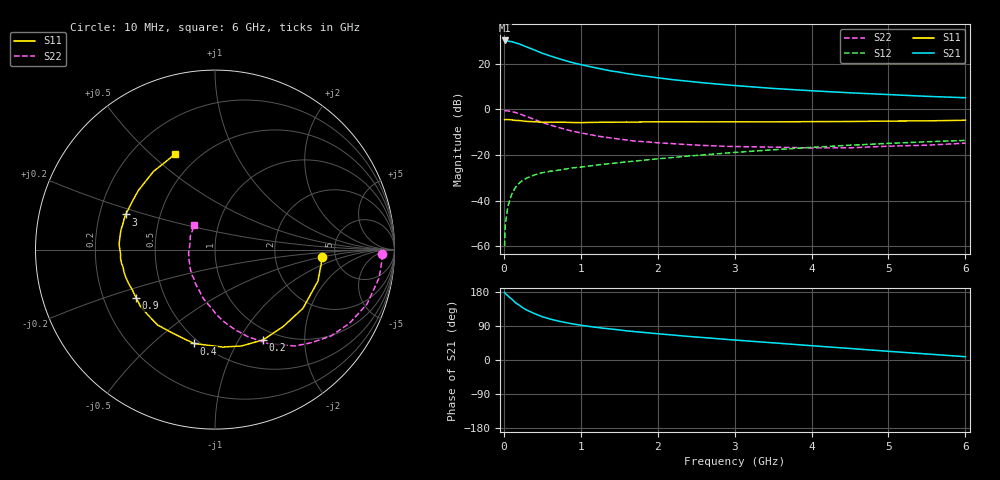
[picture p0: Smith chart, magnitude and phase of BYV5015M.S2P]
! SIEMENS Small Signal Semiconductors
! BFY420
! Si NPN RF SIEGET Grounded Emitter Transistor in MICRO-X
! VCE = 0.5 V  IC = 15 mA
! Common Emitter S-Parameters:  October  1996
# GHz  S  MA  R  50
!  f  S11  S21  S12  S22
! GHz  MAG  ANG  MAG  ANG  MAG  ANG  MAG  ANG
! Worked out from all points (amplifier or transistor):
!   36 points, 10 MHz to 6 GHz, reference 50 ohm
!   highest |S21| = 30.2 dB at 10 MHz (marker M1)
!   |S21| within 3 dB of that: start of sweep to 308.1 MHz
!   unconditionally stable (mu >= 1): start of sweep to 11.19 MHz; 1.834 GHz to end of sweep
!   at 250 MHz: K = 0.27, MSG = 29.5 dB, |S12| = -31.0 dB
!   at 1.4 GHz: K = 0.91, MSG = 20.3 dB, |S12| = -23.7 dB
!   at 6 GHz: K = 1.12, MAG = 7.2 dB, |S12| = -13.6 dB
!   S11 on the Smith chart (normalised r, x): 10 MHz: 3.90, -0.51; 200 MHz: 0.85, -1.27; 400 MHz: 0.47, -0.69; 900 MHz: 0.34, -0.25; 3 GHz: 0.31, +0.17; 6 GHz: 0.37, +0.60
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0.01  0.5979 -4.0  32.53 178.8  0.001 94.5  0.9324 -1.6
0.02  0.5971 -7.4  32.47 175.5  0.003 89.2  0.9322 -3.6
0.05  0.5998 -17.0  31.54 169.8  0.0072 84.0  0.9281 -9.7
0.1  0.5893 -33.8  30.66 161.1  0.0135 76.4  0.8996 -19.7
0.15  0.5727 -48.4  28.92 151.6  0.0194 68.9  0.8545 -28.7
0.2  0.5701 -62.0  27.28 144.6  0.0242 65.1  0.8059 -36.7
0.25  0.5568 -74.7  25.23 137.3  0.0281 59.8  0.7458 -44.1
0.3  0.5448 -85.5  23.31 131.5  0.0314 56.9  0.6972 -50.4
0.4  0.5362 -102.7  20 122.3  0.0367 51.9  0.5977 -60.9
0.5  0.5219 -117.0  17.03 114.2  0.0408 48.8  0.517 -69.5
0.6  0.5279 -127.3  14.95 108.3  0.044 47.0  0.455 -76.5
0.7  0.522 -135.5  13.22 103.1  0.0461 46.3  0.4058 -82.8
0.9  0.5151 -148.6  10.54 95.2  0.0524 45.3  0.3306 -92.8
1.1  0.5174 -158.7  8.829 88.9  0.0569 45.5  0.2843 -102.5
1.4  0.5216 -169.0  6.954 81.6  0.0651 46.1  0.2358 -114.1
1.6  0.5285 -174.8  6.121 76.9  0.0709 45.8  0.2128 -121.7
2.2  0.5343 172.1  4.482 65.8  0.0883 45.0  0.1769 -140.0
3  0.5345 158.5  3.342 52.7  0.1139 41.4  0.1534 -160.5
3.5  0.5332 150.0  2.883 45.3  0.13 38.3  0.1486 -172.3
4.5  0.5427 135.3  2.312 30.4  0.1638 29.8  0.1437 164.6
5.5  0.5607 119.6  1.933 15.9  0.1949 20.0  0.1642 140.4
6  0.5779 112.5  1.802 8.7  0.2092 14.8  0.1817 130.5
